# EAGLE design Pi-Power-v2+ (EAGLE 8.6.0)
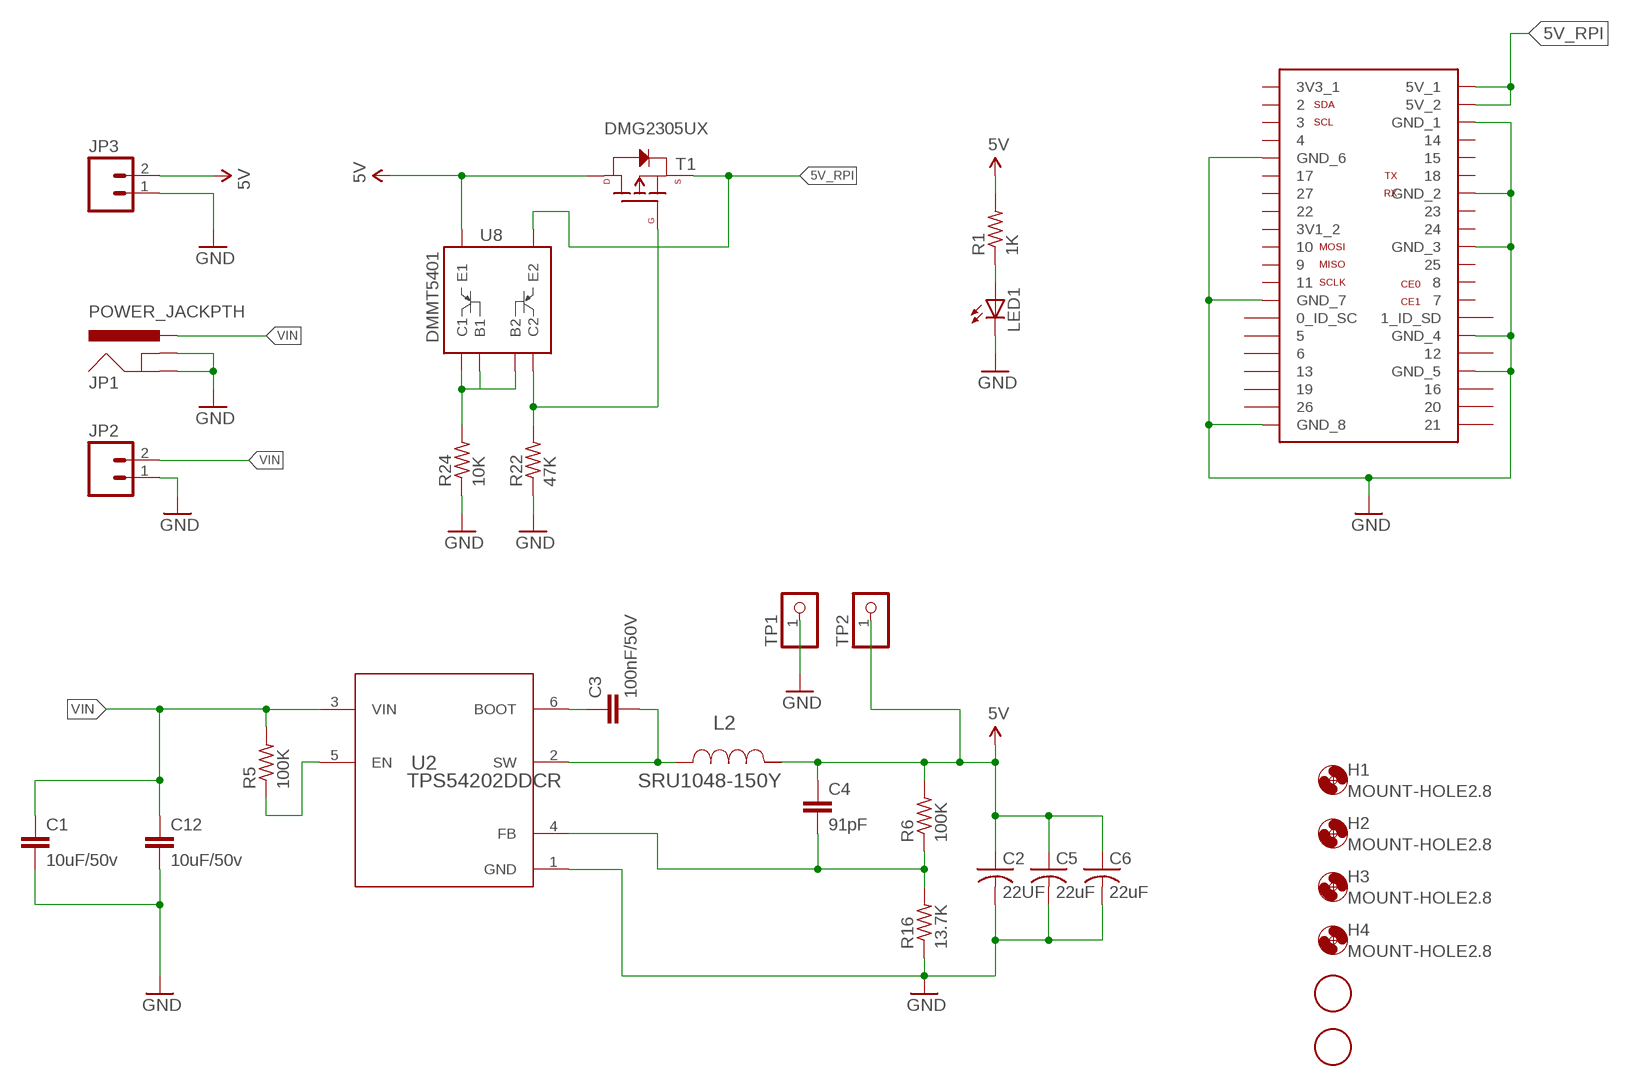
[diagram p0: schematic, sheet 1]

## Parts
C1  10uF/50v  CAP1206  [1206]
C2  22UF  C-USC1210  [C1210]
C3  100nF/50V  CAP0603-CAP  [0603-CAP]
C4  91pF  CAP0603-CAP  [0603-CAP]
C5  22uF  C-USC1210  [C1210]
C6  22uF  C-USC1210  [C1210]
C12  10uF/50v  CAP1206  [1206]
H1  MOUNT-HOLE2.8  [2,8]
H2  MOUNT-HOLE2.8  [2,8]
H3  MOUNT-HOLE2.8  [2,8]
H4  MOUNT-HOLE2.8  [2,8]
JP1  POWER_JACKPTH  [POWER_JACK_PTH]
JP2  M025MM  [SCREWTERMINAL-5MM-2]
JP3  M02PTH  [1X02]
L2  SRU1048-150Y  [SRU1048]
LED1  LEDCHIPLED_0805  [CHIPLED_0805]
R1  1K  R-US_M0805  [M0805]
R5  100K  R-US_R0603  [R0603]
R6  100K  R-US_R0603  [R0603]
R16  13.7K  R-US_R0603  [R0603]
R22  47K  R-US_M0805  [M0805]
R24  10K  R-US_M0805  [M0805]
T1  DMG2305UX  P-CHANNEL-MOSFET  [SOT23-3]
TP1  PINHD-1X1CB  [1X01-CLEANBIG]
TP2  PINHD-1X1CB  [1X01-CLEANBIG]
U1  RASPBERRY-PI-GPIO-SEPARATE  [2X20]
U2  TPS54202DDCR  [DDC0006A_N]
U3  FIDUCIAL  [FIDUCIAL_1MM]
U4  FIDUCIAL  [FIDUCIAL_1MM]
U8  DMMT5401  [SOT-23-6]

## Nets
5V: C2.1 C4.1 C5.1 C6.1 JP3.2 L2.2 R1.2 R6.2 T1.3(D) TP2.1 U8.6(E1)
5V_RPI: T1.2(S) U1.2(5V_1) U1.4(5V_2) U8.5(E2)
GND: C1.2 C2.2 C5.2 C6.2 C12.2 JP1.GND JP1.GNDBREAK JP2.1 JP3.1 LED1.C R16.1 R22.1 R24.1 TP1.1 U1.6(GND_1) U1.9(GND_6) U1.14(GND_2) U1.20(GND_3) U1.25(GND_7) U1.30(GND_4) U1.34(GND_5) U1.39(GND_8) U2.1(GND)
N$1: LED1.A R1.1
N$2: R22.2 T1.1(G) U8.4(C2)
N$5: R5.1 U2.5(EN)
N$7: C4.2 R6.1 R16.2 U2.4(FB)
N$18: C3.2 L2.1 U2.2(SW)
N$20: C3.1 U2.6(BOOT)
N$26: R24.2 U8.1(C1) U8.2(B1) U8.3(B2)
VIN: C1.1 C12.1 JP1.PWR JP2.2 R5.2 U2.3(VIN)
Unconnected: U1.3 U1.5 U1.7 U1.8 U1.10 U1.11 U1.12 U1.13 U1.15 U1.16 U1.18 U1.19 U1.21 U1.22 U1.23 U1.24 U1.26 U1.27(0_ID_SC) U1.28(1_ID_SD) U1.29 U1.31 U1.32 U1.33 U1.35 U1.36 U1.37 U1.38 U1.40

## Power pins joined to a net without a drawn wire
3V1_2: U1.17(3V1_2)
3V3_1: U1.1(3V3_1)

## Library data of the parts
C1 C3 C12 = SparkFun-Capacitors:CAP: Capacitor
C2 C5 C6 = adafruit:C-US: CAPACITOR, American symbol
C4 = SparkFun-Passives:CAP: Capacitor
H1-H4 = holes:MOUNT-HOLE: MOUNTING HOLE with drill center marker
JP1 = SparkFun-Connectors:POWER_JACK: Power Jack This is the standard 5.5mm barrel jack for power. The PTH is the most common, proven, reliable, footprint. The Slot footprint only works if the mill layer is transmitted to the PCB fab house so be warned. Mating wall wart : TOL-00298 (and others); PROD_ID: CONN-08197
JP2 = SparkFun-Connectors:M02: Standard 2-pin 0.1" header. Use with; STOREFRONT_ID: PRT-08432
JP3 = SparkFun-Connectors:M02: Standard 2-pin 0.1" header. Use with
L2 = AlainElements:SRU1048-150Y; DCR: 0.029; IDC: 3.2; L: 1.5E5; MANUFACTURER_NAME: Bourns; MANUFACTURER_PART_NUMBER: SRU1048150Y; VENDOR: Bourns
LED1 = adafruit:LED: LED
R1 R22 R24 = resistor:R-US_: RESISTOR, American symbol
R5 R6 R16 = adafruit:R-US_: RESISTOR, American symbol
T1 = GeekAmmo:P-CHANNEL-MOSFET: P-Channel MOSFET Mode Field Effect Transistor
TP1 TP2 = adafruit:PINHD-1X1: Pin header 1x1 for 0.1" spacing
U1 = pimoroni-headers:RASPBERRY-PI-GPIO-SEPARATE
U2 = AlainElements:TPS54202DDCR; ALTERNATEPARTNUMBER: TPS54202DDCT; APPLICATION_BUILDNUMBER: *; COMPTYPE: IC; MANUFACTURER: Texas Instruments; MANUFACTURER_NAME: Texas Instruments; MANUFACTURER_PART_NUMBER: TPS54202DDCR; MOUNTTYPE: SMT; PACKAGEREFERENCE: DDC0006A; PARTNUMBER: TPS54202DDCR; PIN_COUNT: 6; REFDES: RefDes; ROHS: Y; TYPE: TYPE; VALUE: Value
U3 U4 = adafruit:FIDUCIAL: For use by pick and place machines to calibrate the vision/machine, 1mm
U8 = pimoroni-ics:DMMT5401

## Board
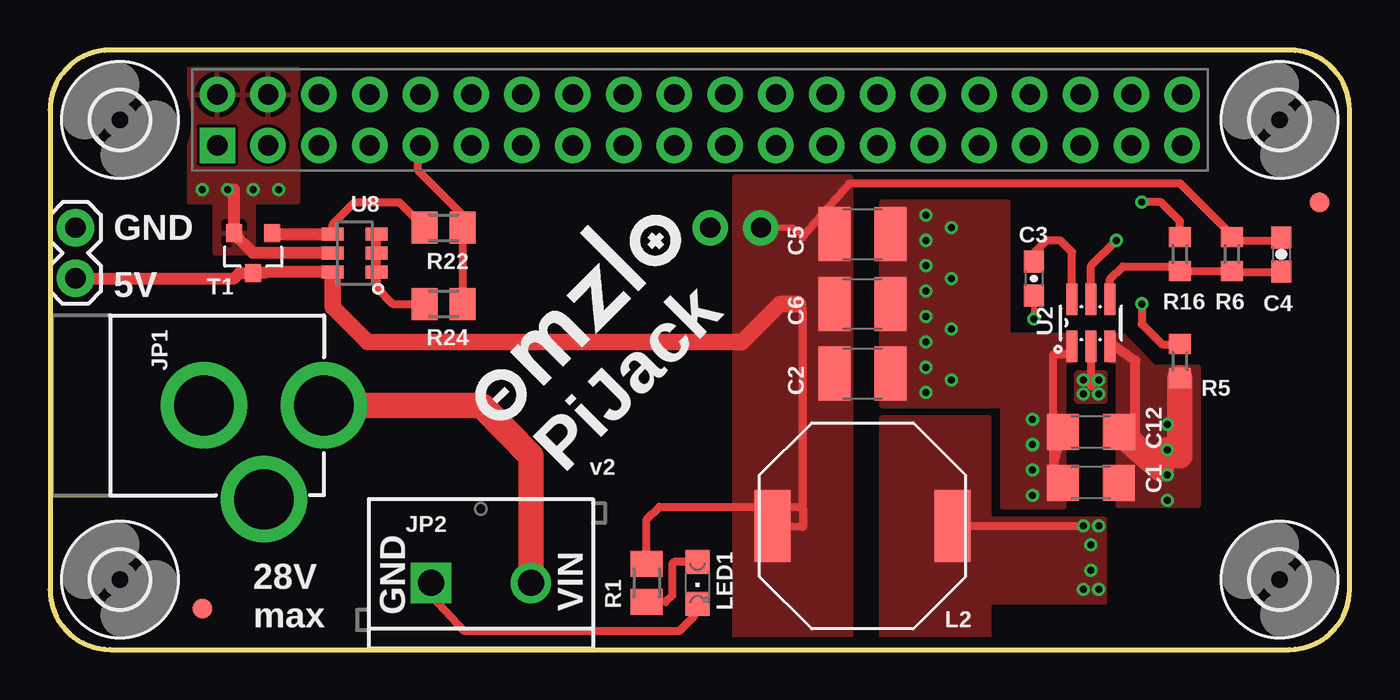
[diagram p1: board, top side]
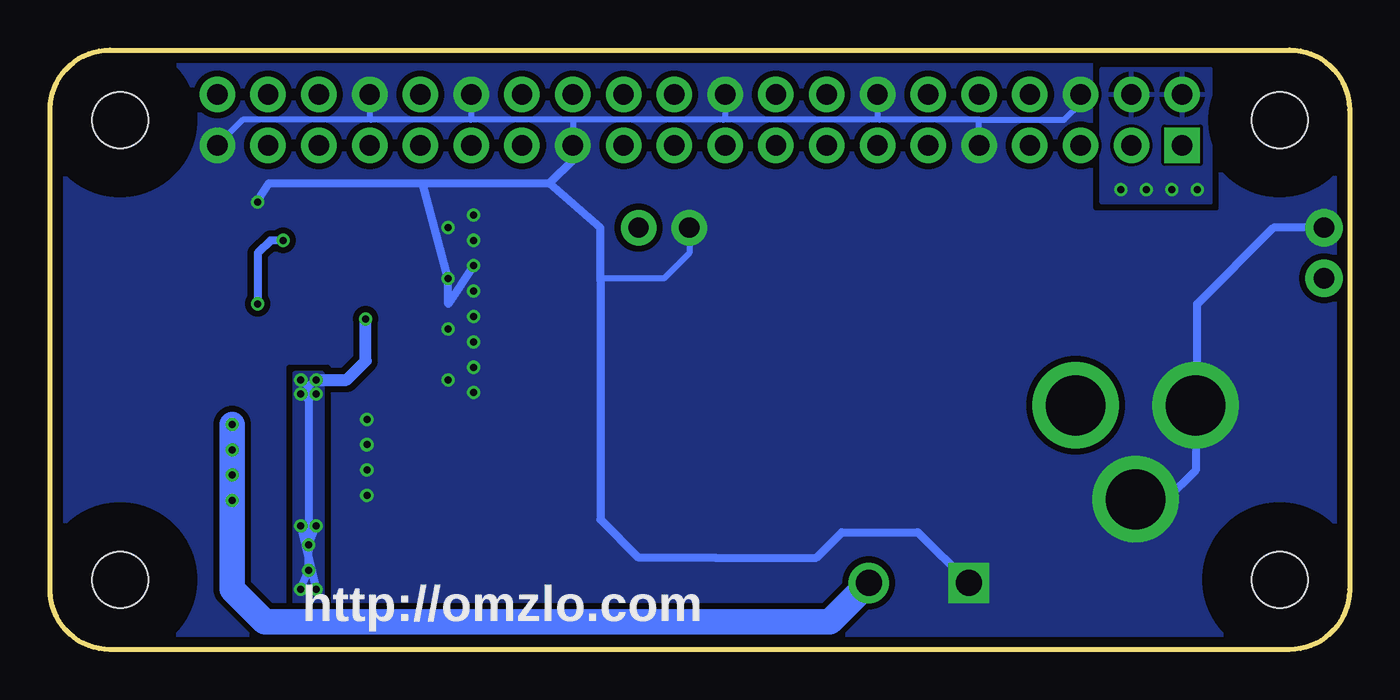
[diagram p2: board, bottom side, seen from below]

Size 65 x 30 mm. Coordinates in mm from the lower left corner, seen from the top.
Outline: 3,30 arc90 0,27 0,3 arc90 3,0 62,0 arc90 65,3 65,27 arc90 62,30 3,30
Copper layers (1*16): Top 0.035mm / dielectric 1.6mm / Bottom 0.035mm
Design rules "Elecrow_2-layer_PCB_eagle_rule": minimum track width 6mil, minimum drill 12mil, track to track 6mil, track to pad 6mil, pad to pad 6mil, via to via 8mil, smd to smd 0mil, copper to edge 20mil, drill to drill 10mil, minimum pad ring 6mil, minimum via ring 6mil, stop-mask expansion 0mil, vias tented up to drill 100mil, thermal gap 10mil

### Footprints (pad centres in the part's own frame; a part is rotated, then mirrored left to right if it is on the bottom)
1206 = smd 1.6 x 1.8: 1 -1.4,0; 2 1.4,0
C1210 = smd 1.6 x 2.7: 1 -1.4,0; 2 1.4,0
0603-CAP = smd 1.1 x 1: 1 -0.85,0; 2 0.85,0
2,8 = hole 2.8: 0,0
POWER_JACK_PTH = drill 2.997 pad 4.318: GND 0,7.7; GNDBREAK 4.7,10.7; PWR 0,13.7
SCREWTERMINAL-5MM-2 = drill 1.3 pad 2.032 square: 1 0,0 | drill 1.3 pad 2.032: 2 5,0
1X02 = drill 1.016 pad 1.88: 1 0,0; 2 2.54,0
SRU1048 = smd 1.803 x 3.607: 1 -4.496,0; 2 4.496,0
CHIPLED_0805 = smd 1.2 x 1.2: A 0,-1.05; C 0,1.05
M0805 = smd 1.3 x 1.6: 1 -0.95,0; 2 0.95,0
R0603 = smd 1 x 1.1: 1 -0.85,0; 2 0.85,0
SOT23-3 = smd 0.8 x 0.9: 1 -0.95,-1; 2 0.95,-1; 3 0,1
1X01-CLEANBIG = drill 1.016 pad 1.778: 1 0,0
2X20 = drill 1.016 pad 1.778 square: 1 -24.13,-1.27 | drill 1.016 pad 1.778: 2 -24.13,1.27; 3 -21.59,-1.27; 4 -21.59,1.27; 5 -19.05,-1.27; 6 -19.05,1.27; 7 -16.51,-1.27; 8 -16.51,1.27; 9 -13.97,-1.27; 10 -13.97,1.27; 11 -11.43,-1.27; 12 -11.43,1.27; 13 -8.89,-1.27; 14 -8.89,1.27; 15 -6.35,-1.27; 16 -6.35,1.27; 17 -3.81,-1.27; 18 -3.81,1.27; 19 -1.27,-1.27; 20 -1.27,1.27; 21 1.27,-1.27; 22 1.27,1.27; 23 3.81,-1.27; 24 3.81,1.27; 25 6.35,-1.27; 26 6.35,1.27; 27 8.89,-1.27; 28 8.89,1.27; 29 11.43,-1.27; 30 11.43,1.27; 31 13.97,-1.27; 32 13.97,1.27; 33 16.51,-1.27; 34 16.51,1.27; 35 19.05,-1.27; 36 19.05,1.27; 37 21.59,-1.27; 38 21.59,1.27; 39 24.13,-1.27; 40 24.13,1.27
DDC0006A_N = smd 1.575 x 0.559: 1 -1.168,0.95; 2 -1.168,0; 3 -1.168,-0.95; 4 1.168,-0.95; 5 1.168,0; 6 1.168,0.95
FIDUCIAL_1MM = smd 1 x 1: 1 0,0
SOT-23-6 = smd 0.65 x 1.1: 1 0.95,1.1; 2 0,1.1; 3 -0.95,1.1; 4 -0.95,-1.1; 5 0,-1.1; 6 0.95,-1.1

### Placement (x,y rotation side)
C1  52.07,8.35 180 top
C2  40.64,13.81 0 top
C3  49.21,18.57 270 top
C4  61.59,19.76 270 top
C5  40.64,17.3 0 top
C6  40.64,20.79 0 top
C12  52.07,10.89 180 top
H1  3.5,26.5 270 top
H2  3.5,3.5 270 top
H3  61.5,26.5 270 top
H4  61.5,3.5 270 top
JP1  0,12.22 270 top
JP2  19.05,3.33 0 top
JP3  1.27,21.11 270 top
L2  40.64,6.19 180 top
LED1  32.38,3.33 180 top
R1  29.84,3.33 90 top
R5  56.52,14.44 270 top
R6  59.12,19.79 90 top
R16  56.52,19.79 270 top
R22  19.68,21.11 180 top
R24  19.68,17.3 180 top
T1  10.16,19.84 180 top
TP1  33.02,21.11 270 top
TP2  35.56,21.11 270 top
U1  32.5,26.5 0 top
U2  52.07,16.35 90 top
U3  7.62,2.06 0 top
U4  63.5,22.38 0 top
U8  15.24,19.84 270 top
U$2  [OMZLO-0.5]  22.54,10.95 45 top

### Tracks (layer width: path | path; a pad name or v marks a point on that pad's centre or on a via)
5V
  Top 0.305: TP2.1 37.19,21.11 37.66,20.63
  Top 0.406: 37.66,7.08 37.66,17.06 37.42,17.3 | 37.66,7.08 37.66,6.12 L2.2 | 37.66,20.63 37.66,20.67 40.01,23.33 56.52,23.33 59.05,20.79 R6.2 59.37,20.47 61.47,20.47 C4.1 | U8.6 | 35.56,16.31 36.86,17.3 | R1.2 29.84,6.51 30.48,7.14 37.6,7.14 37.66,7.08
  Top 0.61: U8.6 10.79,18.89 10.75,18.84 T1.3 9.48,18.84 9.21,18.57 JP3.2 | 14.14,18.46 U8.6
  Top 0.813: 37.42,17.3 36.86,17.3 36.51,17.3 34.61,15.39 15.88,15.39 14.14,17.13 14.14,18.46
  pour Top (no thermals): 34.29,0.16 34.29,23.65 40.01,23.65 40.01,0.16
5V_RPI  (via drill 0.35)
  Top 0.61: U8.5 10.16,19.84 9.21,20.79 T1.2 9.21,23.02 v8.89,23.02
  other vias: 7.62,23.02 10.16,23.02 11.43,23.02
  pour Top: 6.99,22.38 6.99,29.05 12.38,29.05 12.38,22.38 10.16,22.38 10.16,19.84 8.26,19.84 8.26,22.38
  pour Bottom: 12.38,29.05 6.99,29.05 6.99,22.38 12.38,22.38
GND  (via drill 0.35)
  Top 0.406: U2.1 51.12,14.76 50.16,14.76 50.16,9.04 C12.2 | U2.1 | 51.02,14.76 U2.1 | R16.1 56.52,21.43 55.56,22.38 v54.61,22.38 | U1.9 18.41,25.11 18.41,23.97 20.64,21.75 R22.1 R24.1 | JP2.1 19.05,2.69 20.72,0.93 31.47,0.93 32.19,1.65 LED1.C
  Bottom 0.305: U1.6 13.45,27.34 14.29,26.51 18.5,26.51 | 43.95,26.51 48.94,26.51 | 38.81,26.51 43.95,26.51 | 31.32,26.51 38.81,26.51 | 23.51,26.51 31.32,26.51 | 18.5,26.51 23.51,26.51 | 48.94,26.51 55.35,26.51 U1.39 | U1.34 49.01,26.58 48.94,26.51 | U1.30 43.93,26.53 43.95,26.51 | U1.25 38.85,26.47 38.81,26.51 | U1.20 31.23,26.6 31.32,26.51 | U1.14 23.61,26.61 23.51,26.51 | U1.9 18.53,26.48 18.5,26.51 | 31.75,4.62 31.73,4.6 | TP1.1 33.02,19.84 34.29,18.57 37.36,18.57 37.47,18.47
  Bottom 0.406: v54.61,22.38 54.58,22.48 54.05,23.33 46.35,23.33 | 46.35,23.33 40.01,23.33 | 40.01,23.33 37.47,21.11 37.47,18.47 37.47,6.51 35.56,4.6 31.73,4.6 26.67,4.6 25.4,5.87 21.59,5.87 JP2.1 | JP1.GNDBREAK 10.64,7.46 9.21,7.46 7.7,8.96 JP1.GND 7.62,12.3 7.62,17.3 3.81,21.11 JP3.1 | U1.25 38.85,24.49 40.01,23.33 | v43.81,19.2 45.09,17.3 v45.09,18.57 46.35,23.33
  other vias: 43.81,21.75 45.09,21.11 43.81,20.47 43.81,17.93 43.81,14.12 45.09,16.03 43.81,15.39 43.81,12.86 43.81,16.66 49.15,7.71 49.15,8.98 49.15,10.25 49.15,11.52 45.09,13.49
  pour Bottom (isolate 0.305, rank 2, no thermals): 66.04,30 0,30 0,-0.48 66.04,-0.48
  pour Top (no thermals): 41.59,22.38 41.59,12.22 47.62,12.22 47.62,7.14 50.74,7.14 50.74,14.44 51.12,14.44 51.12,15.71 47.94,15.71 47.94,22.38
N$1
  Top 0.406: LED1.A 31.21,4.38 31.11,4.28 31.11,2.69 30.8,2.38 R1.1
N$2
  Top 0.406: U8.4 14.14,21.28 15.24,22.38 17.46,22.38 R22.2
  Top 0.61: T1.1 11.16,20.79 U8.4
N$5  (via drill 0.35)
  Top 0.406: U2.5 52.07,19.2 v53.34,20.47 | v54.61,17.3 54.61,16.28 55.63,15.27 56.39,15.27 R5.1
  Bottom 0.406: v53.34,20.47 53.98,20.47 54.61,19.84 v54.61,17.3
N$7
  Top 0.406: U2.4 53.02,18.53 53.66,19.17 56.2,19.17 56.55,19.02 R16.2 R6.1 59.05,18.89 61.56,18.89 61.61,18.94 C4.2
N$18  (via drill 0.35)
  Top 0.305: C3.2 v49.21,16.55
  Top 0.406: U2.2 52.07,13.17 v52.45,13.49 | L2.1 v51.69,6.19
  Bottom 0.406: 52.07,12.54 52.07,4.92 v52.45,6.19 | v51.69,6.19 51.63,6.19 51.69,6.13 | v51.69,6.19 v52.45,6.19 | 52.1,13.2 52.07,12.54 | 52.1,13.2 v52.45,13.49 | v51.69,13.49 52.12,13.17 52.1,13.2 | v52.45,6.19 v51.69,3.01 v52.45,3.01 v52.07,3.97 v52.07,5.23 51.69,6.13 | v51.69,6.19 51.69,6.13 | v51.69,12.79 52.07,12.54 | v52.45,12.79 52.07,12.54
  Bottom 0.61: v49.21,16.55 49.21,14.44 50.16,13.49 v51.69,13.49
  pour Top (no thermals): 52.77,6.51 46.99,6.51 46.99,11.58 41.59,11.58 41.59,0.16 46.99,0.16 46.99,2.38 52.77,2.38
  pour Top (isolate 0.305): 52.77,13.81 51.37,13.81 51.37,12.47 52.77,12.47
  pour Bottom (isolate 0.305): 52.77,13.81 52.77,2.06 51.37,2.06 51.37,13.81
N$20
  Top 0.406: U2.6 51.12,19.89 50.53,20.47 49.85,20.47 49.21,19.84 C3.1
N$26
  Top 0.406: U8.3 U8.2 U8.1 16.34,18.11 17.14,17.3 R24.2
VIN  (via drill 0.35)
  Top 0.406: JP1.PWR 13.97,12.22
  Top 0.508: C12.1 54.29,9.87 54.29,14.44 53.24,15.18 U2.3
  Top 1.27: 13.97,12.22 21.59,12.22 24.05,9.68 JP2.2 | R5.2 56.52,9.68 v55.88,10 55.56,9.04 C12.1
  Bottom 1.27: JP2.2 25.99,1.39 54.26,1.39 55.88,3.01 v55.88,7.46 v55.88,8.73 v55.88,10 v55.88,11.27
  pour Top (no thermals): 53.02,15.71 53.02,14.44 53.4,14.44 53.4,7.22 57.46,7.22 57.46,14.11 55.24,14.11 54.61,14.76 53.66,15.71

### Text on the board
bPlace: http://omzlo.com
tNames: GND | 5V | PiJack | v2 | VIN | 28V / max | GND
